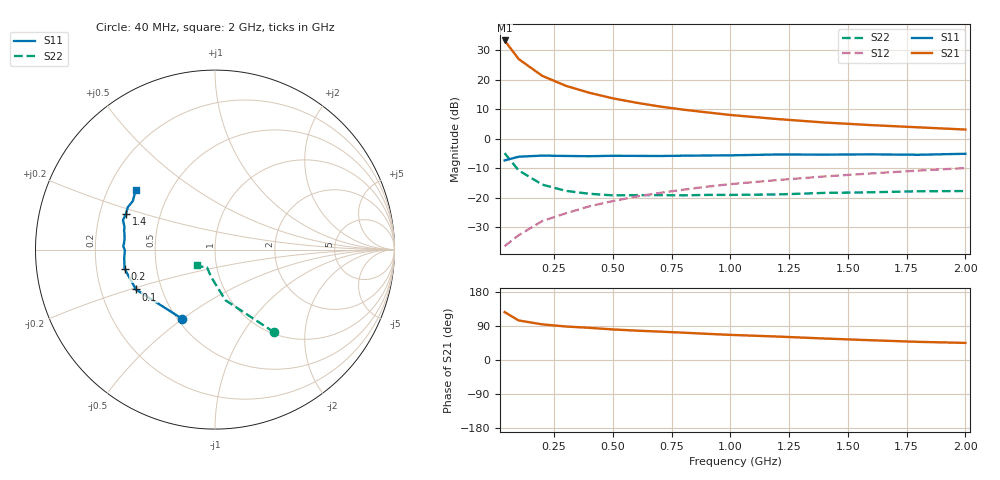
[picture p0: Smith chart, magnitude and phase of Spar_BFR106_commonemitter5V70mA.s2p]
! Filename:  BFR106D.S2P  Version:  2.0
! NXP part #: BFR106  Date: Jun 1990
! Bias condition: Vce=5V, Ic=70mA
#  MHz  S  MA  R  50
! Freq  S11  S21  S12  S22  !GUM [dB]
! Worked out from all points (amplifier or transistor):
!   16 points, 40 MHz to 2 GHz, reference 50 ohm
!   highest |S21| = 33.3 dB at 40 MHz (marker M1)
!   |S21| within 3 dB of that: start of sweep to 68.52 MHz
!   unconditionally stable (mu >= 1): 232.2 MHz to end of sweep
!   at 200 MHz: K = 0.97, MSG = 24.6 dB, |S12| = -28.0 dB
!   at 800 MHz: K = 1.08, MAG = 11.9 dB, |S12| = -17.3 dB
!   at 2 GHz: K = 1.00, MAG = 6.3 dB, |S12| = -10.0 dB
!   S11 on the Smith chart (normalised r, x): 40 MHz: 0.53, -0.50; 100 MHz: 0.36, -0.21; 200 MHz: 0.32, -0.09; 1.4 GHz: 0.31, +0.18; 2 GHz: 0.32, +0.30
40  0.427 -115.1  46.13 126.4  0.015 63.2  0.567 -54.4
100  0.493 -153.2  22.3 104.3  0.023 62.6  0.288 -78.3
200  0.515 -168.0  11.59 94.1  0.04 70.2  0.166 -94.7
300  0.508 -174.8  7.868 88.4  0.054 72.6  0.13 -104.9
400  0.502 -179.5  5.988 84.9  0.071 74.0  0.116 -110.3
500  0.512 177.7  4.82 80.7  0.087 74.2  0.109 -114.6
600  0.509 176.7  4.064 77.5  0.104 74.2  0.11 -116.2
700  0.507 173.6  3.498 74.9  0.12 73.6  0.11 -117.3
800  0.513 169.6  3.094 72.1  0.136 72.8  0.109 -117.6
900  0.517 168.4  2.786 69.1  0.153 72.5  0.111 -117.6
1000  0.52 165.9  2.516 66.3  0.169 71.2  0.111 -119.4
1200  0.538 162.3  2.146 61.9  0.198 69.8  0.113 -123.7
1400  0.535 158.1  1.874 56.7  0.228 68.0  0.12 -127.2
1600  0.54 154.1  1.692 52.1  0.257 66.7  0.123 -129.6
1800  0.532 149.3  1.552 47.9  0.287 64.5  0.128 -133.4
2000  0.553 143.1  1.424 45.1  0.316 63.1  0.129 -139.1
